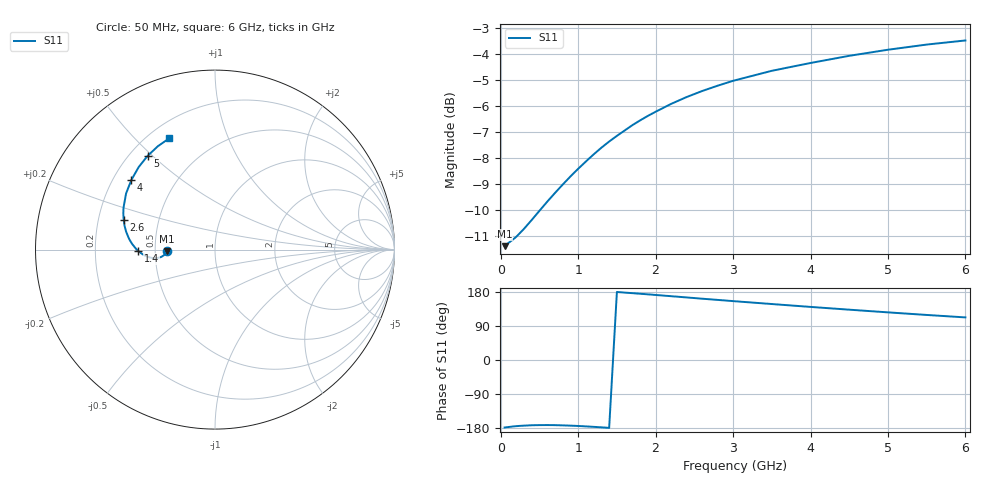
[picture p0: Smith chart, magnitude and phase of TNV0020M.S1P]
! SIEMENS Discrete & RF Semiconductors
! BAS70-07W
! Si Schottky Diode in SOT343
! IF = 20 mA
! S-Parameters:  February  1997
# GHz  S  MA  R  50
!  f  S11
! GHz  MAG  ANG
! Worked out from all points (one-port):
!   34 points, 50 MHz to 6 GHz, reference 50 ohm
!   lowest |S11| = -11.4 dB at 50 MHz (marker M1), VSWR 1.74, Z = 28.8 - j0.526 ohm
!   |S11| at or under -10 dB: start of sweep to 505.9 MHz
!   S11 on the Smith chart (normalised r, x): 50 MHz: 0.58, -0.01; 1.4 GHz: 0.40, -0.01; 2.6 GHz: 0.31, +0.15; 4 GHz: 0.27, +0.34; 5 GHz: 0.27, +0.48; 6 GHz: 0.28, +0.63
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0.05  0.2698 -178.2
0.2  0.2811 -174.6
0.3  0.2912 -173.2
0.4  0.3029 -172.2
0.6  0.3284 -171.7
0.7  0.3413 -171.9
0.8  0.3542 -172.5
0.9  0.3672 -173.2
1  0.3799 -174.1
1.1  0.3924 -175.2
1.3  0.417 -177.7
1.4  0.4286 -179.1
1.5  0.4394 179.5
1.6  0.45 177.9
1.8  0.4706 174.8
1.9  0.48 173.3
2  0.4889 171.6
2.2  0.5062 168.4
2.4  0.5218 165.1
2.6  0.5358 161.8
2.8  0.5486 158.6
3  0.5606 155.4
3.5  0.586 147.7
4  0.6066 140.1
4.5  0.6262 132.8
5  0.6432 125.7
5.5  0.6581 118.9
6  0.6702 112.4
